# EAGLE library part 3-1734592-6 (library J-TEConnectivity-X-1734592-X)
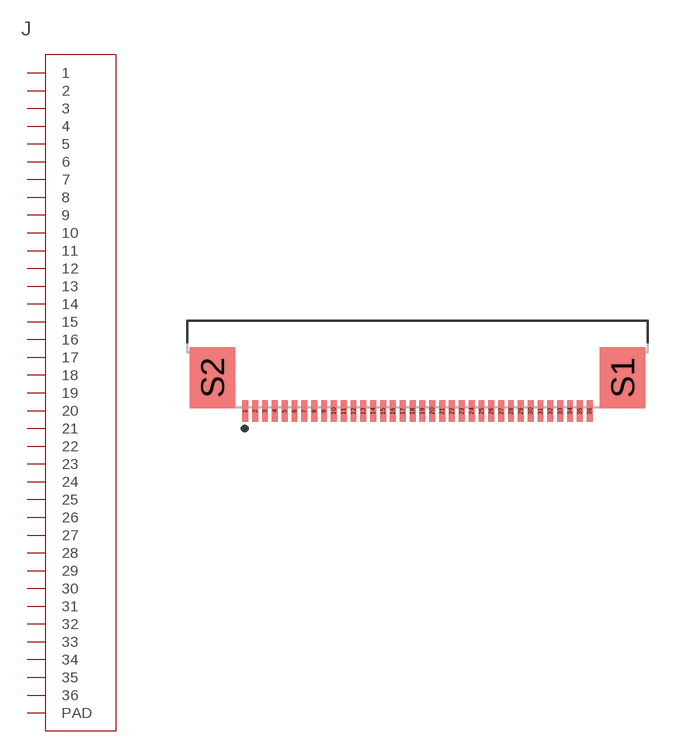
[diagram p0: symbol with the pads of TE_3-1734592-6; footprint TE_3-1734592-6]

Designator prefix J

## 3-1734592-64-1734592-0  [TE_3-1734592-6]
1  1  pas
2  2  pas
3  3  pas
4  4  pas
5  5  pas
6  6  pas
7  7  pas
8  8  pas
9  9  pas
10  10  pas
11  11  pas
12  12  pas
13  13  pas
14  14  pas
15  15  pas
16  16  pas
17  17  pas
18  18  pas
19  19  pas
20  20  pas
21  21  pas
22  22  pas
23  23  pas
24  24  pas
25  25  pas
26  26  pas
27  27  pas
28  28  pas
29  29  pas
30  30  pas
31  31  pas
32  32  pas
33  33  pas
34  34  pas
35  35  pas
36  36  pas
S1  PAD
S2  PAD

## Footprint TE_3-1734592-6 (pad centres in mm)
smd 0.3 x 1.1: 1 -8.75,0; 2 -8.25,0; 3 -7.75,0; 4 -7.25,0; 5 -6.75,0; 6 -6.25,0; 7 -5.75,0; 8 -5.25,0; 9 -4.75,0; 10 -4.25,0; 11 -3.75,0; 12 -3.25,0; 13 -2.75,0; 14 -2.25,0; 15 -1.75,0; 16 -1.25,0; 17 -0.75,0; 18 -0.25,0; 19 0.25,0; 20 0.75,0; 21 1.25,0; 22 1.75,0; 23 2.25,0; 24 2.75,0; 25 3.25,0; 26 3.75,0; 27 4.25,0; 28 4.75,0; 29 5.25,0; 30 5.75,0; 31 6.25,0; 32 6.75,0; 33 7.25,0; 34 7.75,0; 35 8.25,0; 36 8.75,0
smd 2.3 x 3.1: S1 10.42,1.7; S2 -10.42,1.7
